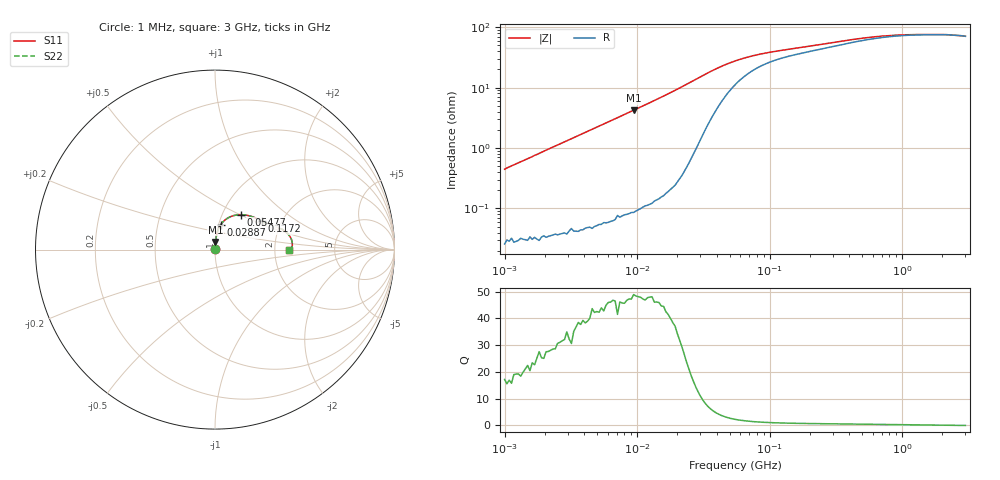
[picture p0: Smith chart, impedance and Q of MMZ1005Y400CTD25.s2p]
! S-Parameter Data Generated by TDK Corporation
! Copyright(C) 2025 TDK Corporation.
! All Rights Reserved.
! TDK P/N: MMZ1005Y400CTD25 (Chip Bead)
! Property: |Z|=40ohm at 100MHz
! Size(LxWxT): 1x0.5x0.5mm
! Model Type: s2p (Touchstone File Format Version 1.0)
! Frequency: DC=Yes Start=1MHz Stop=3000MHz 202points Log-sweep
! Model Generated on Feb. 6, 2025
! Terms and conditions regarding TDK Simulation Models:
! 1)This simulation model is being provided solely for informational
!  purposes. Please refer to the specifications of the products in
!  terms of detailed characteristics of such products.
! 2)In no event shall TDK Corporation of any of its subsidiaries be
!  liable for any loss or damage arising, directly or indirectly,
!  from any information contained in this simulation model, including,
!  but not limited to loss or damages arising from any inaccuracies,
!  omissions or errors in connection with such information.
! 3)Any and all copyrights on this simulation model are owned by
!  TDK Corporation.  Duplication or redistribution of this simulation
!  model without prior written permission from TDK Corporation
!  is prohibited.
! 4)This simulation model is subject to any modification or change
!  without any prior notice.
! 5)Neither TDK Corporation nor any of its subsidiaries shall make any
!  warranty, express or implied, including but not limited to the
!  correctness, implied warranties of merchantability and fitness for
!  a particular purpose with respect to this simulation models.
! 6)The use of this simulation model shall be deemed to have consented
!  to the terms and conditions hereof.
! Port Assignments:
!  1 ---@@@--- 2
! Applicable Conditions:
!  Temperature = 25 degC
!  DC Bias Current = 0 A
!  Small Signal Operation
# Hz S MA R 50
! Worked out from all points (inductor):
!   201 points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, 1 MHz to 3 GHz, reference 50 ohm
!   read as one part in series: L = 71.4 nH near 1.041 MHz
!   highest Q = 48.2 at 9.41 MHz (marker M1), where L = 71.3 nH
!   self-resonance near 2.849 GHz
!   S11 on the Smith chart (normalised r, x): 1 MHz: 1.00, +0.01; 28.87 MHz: 1.02, +0.29; 54.77 MHz: 1.22, +0.51; 117.2 MHz: 1.59, +0.56; 3 GHz: 2.42, -0.02
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1000000  0.004462 86.4  0.9997 -0.3  0.9997 -0.3  0.004462 86.4
1127605  0.005088 86.1  0.9997 -0.3  0.9997 -0.3  0.005088 86.1
1616692  0.007215 87.1  0.9997 -0.4  0.9997 -0.4  0.007215 87.1
3900413  0.0174 87.5  0.9994 -1.0  0.9994 -1.0  0.0174 87.5
9410094  0.04211 86.4  0.9983 -2.4  0.9983 -2.4  0.04211 86.4
1.461624e7  0.0663 85.0  0.9964 -3.8  0.9964 -3.8  0.0663 85.0
2.095589e7  0.09809 82.6  0.9921 -5.6  0.9921 -5.6  0.09809 82.6
2.886629e7  0.1412 77.3  0.9788 -8.1  0.9788 -8.1  0.1412 77.3
3.387922e7  0.1675 72.7  0.9635 -9.6  0.9635 -9.6  0.1675 72.7
3.976269e7  0.1945 66.8  0.9405 -11.0  0.9405 -11.0  0.1945 66.8
4.666789e7  0.2201 60.2  0.9107 -12.1  0.9107 -12.1  0.2201 60.2
5.477226e7  0.2422 53.4  0.8775 -12.8  0.8775 -12.8  0.2422 53.4
6.428402e7  0.2608 47.2  0.8449 -13.1  0.8449 -13.1  0.2608 47.2
7.852918e7  0.2795 40.6  0.8083 -13.0  0.8083 -13.0  0.2795 40.6
1.171891e8  0.3069 31.0  0.7536 -12.1  0.7536 -12.1  0.3069 31.0
2.136344e8  0.3449 23.1  0.6962 -11.2  0.6962 -11.2  0.3449 23.1
4.391493e8  0.3971 15.8  0.6272 -9.9  0.6272 -9.9  0.3971 15.8
8.005644e8  0.4252 9.5  0.5849 -6.9  0.5849 -6.9  0.4252 9.5
1.147801e9  0.4314 6.4  0.5733 -4.8  0.5733 -4.8  0.4314 6.4
1.855641e9  0.4317 3.2  0.5695 -2.5  0.5695 -2.5  0.4317 3.2
2.556106e9  0.4242 1.0  0.5759 -0.7  0.5759 -0.7  0.4242 1.0
3e9  0.4146 -0.4  0.5854 0.3  0.5854 0.3  0.4146 -0.4
